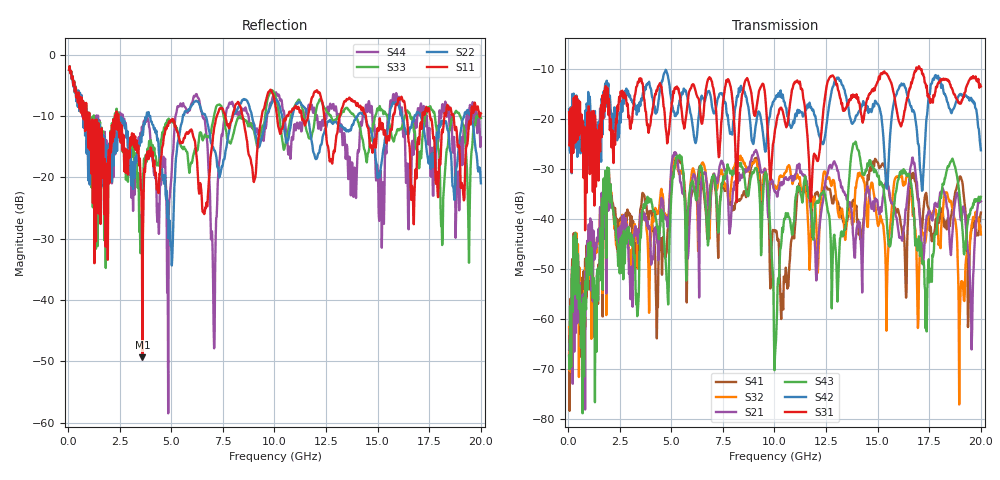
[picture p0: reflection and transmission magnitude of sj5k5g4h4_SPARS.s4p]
! FILE: E:\users\goganessyan\GBX_Backplane\FR408_backplane\1m_OUTBOUND_NEXT\sj5k5g4h4_SPARS.s4p
# MHZ S RI R 50.00
! FREQ  S11  S12  S13  S14
!  S21  S22  S23  S24
!  S31  S32  S33  S34
!  S41  S42  S43  S44
!  REAL  IMAG  REAL  IMAG  REAL  IMAG  REAL  IMAG
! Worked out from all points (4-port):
!   799 points, 50 MHz to 20 GHz, reference 50 ohm
!   strongest paths, dB at 50 MHz, 5.025 GHz, 10.03 GHz, 15.03 GHz, 20 GHz:
!     S31: -18.6, -16.7, -22.1, -12.3, -13.5
!     S42: -18.0, -17.0, -16.0, -17.1, -26.2
!     S43: -67.3, -34.1, -67.2, -31.4, -35.5
!     S21: -66.0, -28.7, -34.6, -38.1, -36.4
!     S32: -61.6, -29.9, -33.3, -41.4, -43.1
!     S41: -66.9, -32.4, -42.3, -28.9, -38.7
!   lowest |S11| = -49.3 dB at 3.6 GHz (marker M1), VSWR 1.01, Z = 49.7 + j0.0948 ohm
!   |S11| at or under -10 dB: 1.027 GHz to 2.274 GHz (1.247 GHz wide, 75.5 % of centre); 2.433 GHz to 7.207 GHz (4.774 GHz wide, 99.1 % of centre); 14.43 GHz to 15.75 GHz (1.319 GHz wide, 8.75 % of centre)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
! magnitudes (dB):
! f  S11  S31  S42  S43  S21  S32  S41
! 50 MHz  -2.5  -18.6  -18.0  -67.3  -66.0  -61.6  -66.9
! 3.6 GHz  -49.3  -12.8  -15.7  -38.3  -38.5  -39.9  -34.8
! 7.075 GHz  -12.0  -14.9  -18.9  -31.6  -30.9  -31.5  -32.3
! 9.575 GHz  -7.6  -16.7  -26.5  -30.6  -30.7  -30.3  -30.8
! 10.05 GHz  -8.4  -21.7  -16.0  -65.7  -34.5  -33.6  -42.6
! 13.9 GHz  -7.6  -15.5  -20.1  -24.8  -47.7  -35.4  -37.5
! 20 GHz  -9.6  -13.5  -26.2  -35.5  -36.4  -43.1  -38.7
